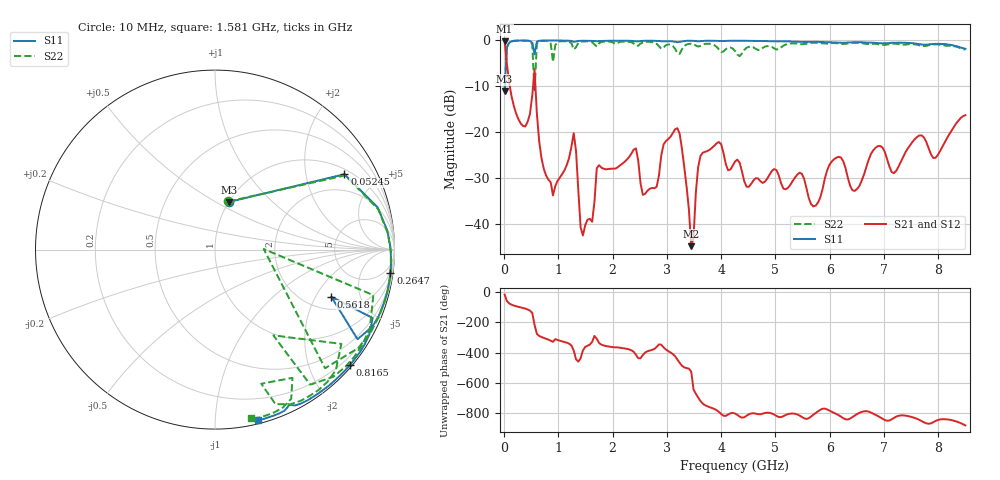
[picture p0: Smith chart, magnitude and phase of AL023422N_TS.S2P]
!AVX CORPORATION
!PN: AL023422N_TS
!DESCRIPTION: AIR CORE INDUCTOR, 422nH, 18 turns
!Agilent Technologies,E5071C,MY46102230,A.09.54
!Date: Mon Sep 03 16:49:50 2012
!Data & Calibration Information:
!Freq	S11:SOLT2(ON)	S21:SOLT2(ON)	S12:SOLT2(ON)	S22:SOLT2(ON)
# Hz S dB R 50
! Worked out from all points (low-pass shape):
!   201 points, 10 MHz to 8.5 GHz, reference 50 ohm
!   highest |S21| = -0.32 dB at 10 MHz (marker M1); lowest = -44.9 dB at 3.448 GHz (marker M2)
!   |S21| within 3 dB of the highest: start of sweep to 35.92 MHz
!   lowest |S11| = -11.2 dB at 10 MHz (marker M3), VSWR 1.76, Z = 50.1 + j28.8 ohm
!   |S11| at or under -10 dB: start of sweep to 15.19 MHz
!   |S22| runs from -11.3 to -0.1 dB; largest |S21 - S12| = 0.0028
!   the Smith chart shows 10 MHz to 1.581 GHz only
!   S11 on the Smith chart (normalised r, x): 10 MHz: 1.00, +0.58; 52.45 MHz: 1.20, +3.30; 264.7 MHz: 2, -15; 561.9 MHz: 2.65, -2.72; 816.5 MHz: 0.04, -2.70; 1.581 GHz: 0.03, -1.28
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1e7  -11.17 73.8  -0.32 -16.8  -0.29 -16.7  -11.10 74.4
5.245e7  -1.57 30.2  -5.23 -59.8  -5.21 -59.9  -1.56 29.7
2.647e8  -0.12 -7.6  -17.25 -98.2  -17.23 -98.3  -0.11 -9.8
5.194e8  -0.56 -32.2  -12.06 -138.1  -12.06 -138.2  -0.90 -47.2
5.6185e8  -3.11 -22.1  -6.42 143.6  -6.41 143.6  -11.32 0.7
6.043e8  -0.38 -23.5  -15.98 83.6  -15.98 83.5  -0.74 -16.1
8.1655e8  -0.09 -40.6  -30.39 45.6  -30.37 45.8  -0.29 -47.2
1.2835e9  -0.39 -64.6  -20.27 -26.5  -20.27 -26.4  -2.04 -71.0
1.4533e9  -0.17 -70.6  -42.53 -25.5  -42.55 -25.7  -0.31 -69.9
1.58065e9  -0.18 -75.8  -38.91 12.6  -39.03 12.8  -0.35 -78.0
1.75045e9  -0.22 -81.6  -27.23 23.5  -27.28 23.3  -0.72 -79.1
2.85415e9  -0.22 -112.1  -29.45 14.0  -29.46 14.0  -1.34 -119.1
3.19375e9  -0.47 -118.2  -19.19 -86.3  -19.20 -86.2  -2.85 -121.8
3.44845e9  -0.17 -113.2  -44.86 -166.0  -44.76 -165.6  -0.81 -117.7
3.61825e9  -0.25 -114.0  -25.25 0.2  -25.26 0.2  -1.29 -120.6
4.255e9  -0.17 -120.0  -26.45 -82.1  -26.43 -82.1  -2.39 -140.9
5.6983e9  -0.39 -141.7  -36.22 -90.2  -36.17 -90.9  -0.61 -157.1
6.1228e9  -0.51 -149.9  -25.60 -85.2  -25.63 -85.1  -0.69 -162.9
6.4624e9  -0.48 -155.2  -32.83 -94.6  -32.92 -94.2  -0.59 -164.8
6.84445e9  -0.61 -162.8  -23.45 -90.9  -23.43 -90.8  -0.83 -167.0
7.09915e9  -0.66 -166.1  -27.51 -128.5  -27.55 -128.5  -0.88 -165.9
8.5e9  -1.90 168.0  -16.36 -161.1  -16.37 -161.2  -2.12 -172.2
